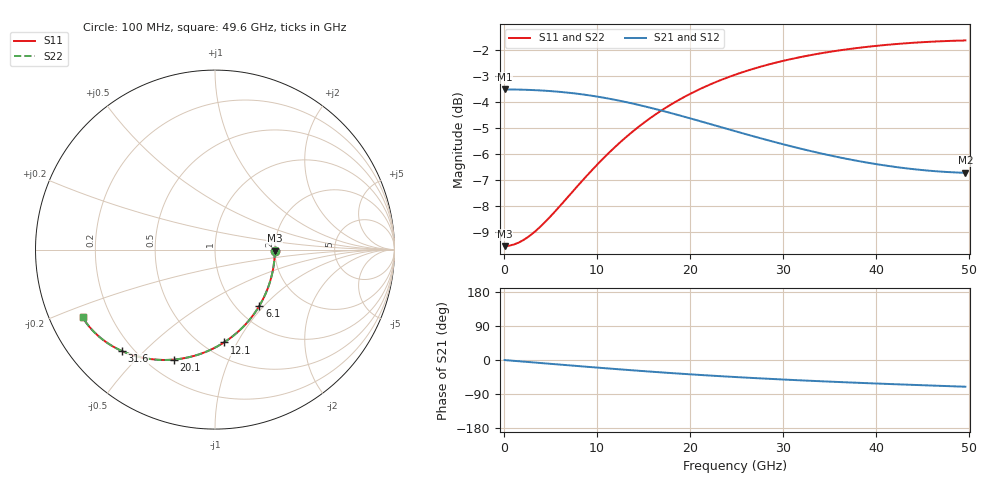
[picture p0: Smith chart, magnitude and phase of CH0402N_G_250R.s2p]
# GHz S RI R 250
! S-Parameters data
! Freq  reS11  imS11  reS21  imS21  reS12  imS12  reS22  imS22
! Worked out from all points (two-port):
!   100 points, 100 MHz to 49.6 GHz, reference 250 ohm
!   highest |S21| = -3.52 dB at 100 MHz (marker M1); lowest = -6.7 dB at 49.6 GHz (marker M2)
!   |S21| within 3 dB of the highest: start of sweep to 42.57 GHz
!   lowest |S11| = -9.5 dB at 100 MHz (marker M3), VSWR 2.00, Z = 500 - j6.21 ohm
!   |S11| at or under -10 dB: nowhere
!   |S22| runs from -9.5 to -1.6 dB; largest |S21 - S12| = 0
!   S11 on the Smith chart (normalised r, x): 100 MHz: 2.00, -0.02; 6.1 GHz: 1.26, -0.94; 12.1 GHz: 0.62, -0.88; 20.1 GHz: 0.30, -0.65; 31.6 GHz: 0.16, -0.43; 49.6 GHz: 0.10, -0.24
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0.1  0.3333 -0.00552  0.6667 -0.00233  0.6667 -0.00233  0.3333 -0.00552
1.6  0.327 -0.0879  0.6652 -0.0372  0.6652 -0.0372  0.327 -0.0879
3.1  0.3098 -0.168  0.661 -0.0719  0.661 -0.0719  0.3098 -0.168
4.6  0.2827 -0.2438  0.6541 -0.1061  0.6541 -0.1061  0.2827 -0.2438
6.1  0.247 -0.3136  0.6445 -0.1395  0.6445 -0.1395  0.247 -0.3136
7.6  0.2042 -0.3763  0.6322 -0.1718  0.6322 -0.1718  0.2042 -0.3763
8.6  0.1726 -0.4138  0.6226 -0.1925  0.6226 -0.1925  0.1726 -0.4138
10.1  0.1219 -0.4634  0.6063 -0.222  0.6063 -0.222  0.1219 -0.4634
12.1  0.0503 -0.5171  0.5813 -0.2582  0.5813 -0.2582  0.0503 -0.5171
14.1  -0.0228 -0.5574  0.5535 -0.2902  0.5535 -0.2902  -0.0228 -0.5574
16.6  -0.1127 -0.5911  0.5163 -0.3239  0.5163 -0.3239  -0.1127 -0.5911
18.1  -0.1646 -0.6036  0.4933 -0.3408  0.4933 -0.3408  -0.1646 -0.6036
20.1  -0.2304 -0.6128  0.4627 -0.3599  0.4627 -0.3599  -0.2304 -0.6128
22.6  -0.3064 -0.6144  0.4252 -0.3786  0.4252 -0.3786  -0.3064 -0.6144
25.1  -0.375 -0.6075  0.3894 -0.3924  0.3894 -0.3924  -0.375 -0.6075
28.1  -0.4476 -0.5911  0.3495 -0.4041  0.3495 -0.4041  -0.4476 -0.5911
31.6  -0.52 -0.5644  0.3074 -0.4128  0.3074 -0.4128  -0.52 -0.5644
33.1  -0.5472 -0.5512  0.2908 -0.4154  0.2908 -0.4154  -0.5472 -0.5512
37.1  -0.6102 -0.5127  0.2507 -0.4204  0.2507 -0.4204  -0.6102 -0.5127
41.6  -0.6666 -0.4659  0.2117 -0.4247  0.2117 -0.4247  -0.6666 -0.4659
45.6  -0.7059 -0.4225  0.1814 -0.4289  0.1814 -0.4289  -0.7059 -0.4225
49.6  -0.7366 -0.3779  0.1538 -0.4347  0.1538 -0.4347  -0.7366 -0.3779
